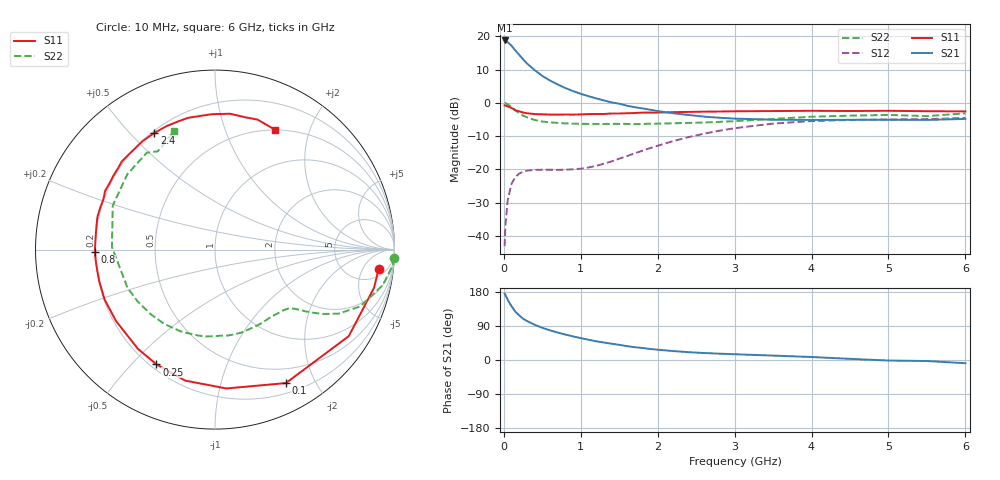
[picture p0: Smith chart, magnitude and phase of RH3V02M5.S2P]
! SIEMENS Small Signal Semiconductors
! BFR106
! Si NPN RF Bipolar Junction Transistor in SOT23
! VCE = 3 V  IC = 2.5 mA
! Common Emitter S-Parameters:  August  1996
# GHz  S  MA  R  50
!  f  S11  S21  S12  S22
! GHz  MAG  ANG  MAG  ANG  MAG  ANG  MAG  ANG
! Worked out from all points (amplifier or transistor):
!   36 points, 10 MHz to 6 GHz, reference 50 ohm
!   highest |S21| = 18.8 dB at 10 MHz (marker M1)
!   |S21| within 3 dB of that: start of sweep to 149.5 MHz
!   unconditionally stable (mu >= 1): 744.7 MHz to 2.032 GHz; 3.91 GHz to end of sweep
!   at 250 MHz: K = 0.36, MSG = 16.9 dB, |S12| = -20.7 dB
!   at 1.4 GHz: K = 1.23, MAG = 6.0 dB, |S12| = -17.6 dB
!   at 6 GHz: K = 1.02, MAG = -1.0 dB, |S12| = -4.5 dB
!   S11 on the Smith chart (normalised r, x): 10 MHz: 8, -11; 100 MHz: 0.32, -1.62; 250 MHz: 0.22, -0.59; 800 MHz: 0.20, -0.01; 2.4 GHz: 0.21, +0.59; 6 GHz: 0.50, +1.50
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0.01  0.9176 -6.9  8.711 175.1  0.007 86.0  0.9978 -2.6
0.02  0.9117 -13.4  8.612 171.6  0.0142 81.7  0.9941 -5.1
0.05  0.8877 -32.9  8.205 158.7  0.0344 71.9  0.9552 -12.0
0.1  0.8422 -62.0  7.26 142.0  0.0608 58.4  0.8686 -21.4
0.15  0.7763 -85.3  6.157 127.5  0.0771 47.2  0.7752 -27.4
0.2  0.7485 -102.8  5.293 117.7  0.0864 40.3  0.7027 -30.7
0.25  0.718 -117.0  4.522 109.1  0.0921 35.1  0.6443 -33.0
0.3  0.6999 -127.9  3.929 103.0  0.0956 32.1  0.6078 -34.4
0.4  0.68 -144.3  3.121 93.1  0.0983 28.4  0.554 -36.5
0.5  0.6751 -155.7  2.548 85.0  0.0989 27.4  0.5252 -38.6
0.6  0.6684 -165.1  2.174 78.2  0.099 28.3  0.5103 -41.3
0.8  0.6699 -178.8  1.676 67.1  0.0991 33.4  0.4929 -47.7
1.1  0.68 164.4  1.264 53.4  0.1068 46.1  0.4843 -59.2
1.6  0.6997 144.0  0.908 36.6  0.1583 62.6  0.4839 -81.7
2.2  0.7267 123.6  0.7 23.6  0.2664 62.4  0.4942 -112.4
2.4  0.7326 117.4  0.659 20.6  0.3061 59.4  0.5012 -124.1
3  0.7494 101.5  0.581 15.2  0.417 47.2  0.532 -156.5
3.5  0.7547 91.3  0.559 11.6  0.4889 35.8  0.5744 178.5
4.5  0.7561 77.3  0.557 3.0  0.5545 15.0  0.6441 139.3
5  0.7618 71.9  0.558 -1.4  0.5654 7.1  0.6599 125.1
5.5  0.751 66.6  0.555 -2.7  0.5713 3.3  0.6333 120.2
6  0.7467 63.4  0.575 -8.5  0.5945 -4.4  0.6972 109.2
